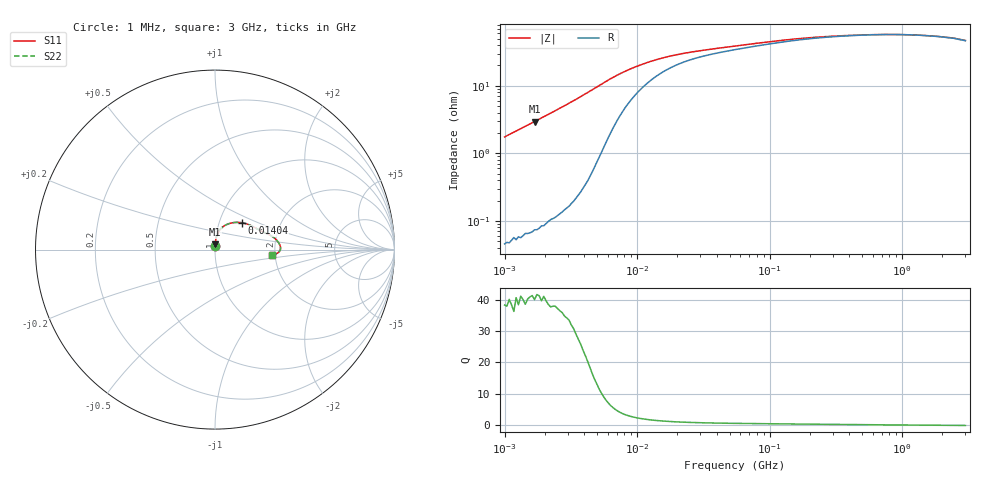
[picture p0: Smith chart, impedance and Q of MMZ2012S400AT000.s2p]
! S-parameter Generated by TDK Corporation
! Copyright(C) 2016 TDK Corporation.
! All Rights Reserved.
! TDK P/N: MMZ2012S400AT000 (Chip Beads)
! Property: |Z|=40¶ at 100MHz
! Size(LxWxT): 2x1.25x0.85mm, 0.079x0.049x0.033inches
! Model Type: s2p (Touchstone File Format Version 1.0)
! Frequency: DC=Yes Start=1MHz Stop=3000MHz 202points Log-sweep
! Note: This model was converted from impedance.
! Model Generated on May. 16, 2016
! Hash(MD5):
! Port Assignments:
!  1 ---@@@--- 2
! Applicable Conditions:
!  Temperature = 25 degC
!  DC Bias Current = 0 A
!  Small Signal Operation
! Terms and conditions regarding TDK Simulation Models
! (1)This simulation model is being provided solely for informational purposes. Please refer to the specifications of the products in terms of detailed characteristics of such products.
! (2)In no event shall TDK Corporation of any of its subsidiaries be liable for any loss or damage arising, directly or indirectly,
!  From any information contained in this simulation model, including, but not limited to loss or damages arising from any inaccuracies, omissions or errors in connection with such information.
! (3)Any and all copyrights on this simulation model are owned by TDK Corporation.
!  Duplication or redistribution of this simulation model without prior written permission from TDK Corporation is prohibited.
! (4)This simulation model is subject to any modification or change without any prior notice.
! (5)Neither TDK Corporation nor any of its subsidiaries shall make any warranty, express or implied,
!  Including but not limited to the correctness, implied warranties of merchantability and fitness for a particular purpose with respect to this simulation models.
! (6)The use of this simulation model shall be deemed to have consented to the terms and conditions hereof.
# MHz S MA R 50
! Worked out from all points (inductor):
!   201 points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, 1 MHz to 3 GHz, reference 50 ohm
!   read as one part in series: L = 279 nH near 1.041 MHz
!   highest Q = 41.3 at 1.683 MHz (marker M1), where L = 279 nH
!   self-resonance near 1.032 GHz
!   S11 on the Smith chart (normalised r, x): 1 MHz: 1.00, +0.03; 14.04 MHz: 1.28, +0.40; 3 GHz: 1.93, -0.13
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1  0.01743 87.5  0.9994 -1.0  0.9994 -1.0  0.01743 87.5
1.682724  0.02951 86.9  0.9988 -1.7  0.9988 -1.7  0.02951 86.9
2.511129  0.04452 85.9  0.9978 -2.6  0.9978 -2.6  0.04452 85.9
3.900413  0.07186 83.5  0.9944 -4.1  0.9944 -4.1  0.07186 83.5
4.959344  0.09496 80.2  0.9883 -5.4  0.9883 -5.4  0.09496 80.2
5.820586  0.1138 76.4  0.9794 -6.5  0.9794 -6.5  0.1138 76.4
7.400828  0.1438 68.2  0.956 -8.0  0.956 -8.0  0.1438 68.2
8.686058  0.1628 62.2  0.9351 -8.9  0.9351 -8.9  0.1628 62.2
10.19448  0.1806 56.2  0.9119 -9.5  0.9119 -9.5  0.1806 56.2
14.04268  0.2113 45.1  0.864 -10.0  0.864 -10.0  0.2113 45.1
14.61624  0.2146 43.9  0.8583 -10.0  0.8583 -10.0  0.2146 43.9
17.85516  0.2296 38.1  0.8316 -9.8  0.8316 -9.8  0.2296 38.1
23.62996  0.2464 31.6  0.8006 -9.3  0.8006 -9.3  0.2464 31.6
54.77226  0.2863 20.1  0.7377 -7.7  0.7377 -7.7  0.2863 20.1
121.9755  0.324 13.5  0.6892 -6.3  0.6892 -6.3  0.324 13.5
213.6344  0.3447 9.4  0.6623 -4.9  0.6623 -4.9  0.3447 9.4
405.36  0.3592 5.3  0.6432 -3.0  0.6432 -3.0  0.3592 5.3
800.5644  0.3655 1.4  0.6347 -0.8  0.6347 -0.8  0.3655 1.4
1194.682  0.362 -0.8  0.638 0.5  0.638 0.5  0.362 -0.8
1782.824  0.352 -2.8  0.6486 1.5  0.6486 1.5  0.352 -2.8
2455.801  0.3376 -4.5  0.664 2.3  0.664 2.3  0.3376 -4.5
3000  0.32 -5.5  0.6822 2.6  0.6822 2.6  0.32 -5.5
